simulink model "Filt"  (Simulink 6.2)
settings: Solver=ode45  StartTime=0.0  StopTime=10.0  RelTol=1e-3
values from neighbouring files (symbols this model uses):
  wd = 7    [run.m]    (also in run3.m)
  wd2 = 16    [run.m]    (also in run3.m)
  wf = 9    [run.m]    (also in run3.m)
  wn = 7.4    [run.m]    (also in run3.m)
  wn2 = 16.8    [run.m]    (also in run3.m)
  zd = 0.2    [run.m]    (also in run3.m)
  zd2 = 0.2    [run.m]    (also in run3.m)
  zn = 0.02    [run.m]    (also in run3.m)
  zn2 = 0.015    [run.m]    (also in run3.m)

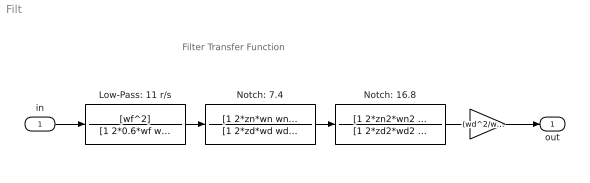
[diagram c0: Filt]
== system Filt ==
  note: Filter Transfer Function
  in : Inport  Port=1  LatchInput=off
  " " : Gain  Gain=(wd^2/wn^2)*(wd2^2/wn2^2)
  Low-Pass: 11 r/s : TransferFcn  Numerator=[wf^2]  Denominator=[1 2*0.6*wf wf^2]
  Notch: 16.8 : TransferFcn  Numerator=[1 2*zn2*wn2 wn2^2]  Denominator=[1 2*zd2*wd2 wd2^2]
  Notch: 7.4 : TransferFcn  Numerator=[1 2*zn*wn wn^2]  Denominator=[1 2*zd*wd wd^2]
  out : Outport
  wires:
  in/1 -> Low-Pass: 11 r/s/1
  Notch: 7.4/1 -> Notch: 16.8/1
  Notch: 16.8/1 -> " "/1
  " "/1 -> out/1
  Low-Pass: 11 r/s/1 -> Notch: 7.4/1
